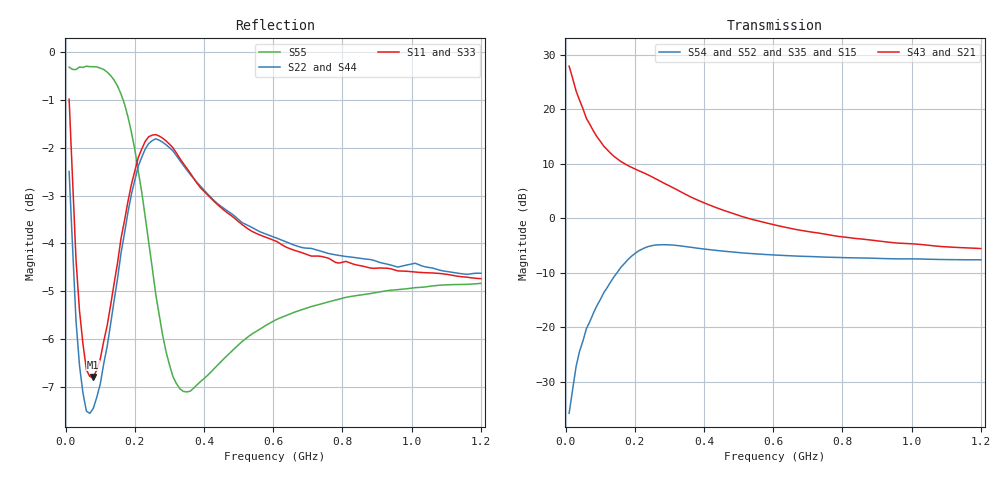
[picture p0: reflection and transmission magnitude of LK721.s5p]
! Date: Fri Jan 15 13:51:43 1999
!  POLYFET RF DEVICES
!  LK721 (EACH SIDE)
!  12.5Vdc		200ma
!AWR Design Environment (2053) Wed Feb 04 14:52:41 2004
!freq-unit  param-type  data-format  keyword  impedance-ohms
# MHz  S  MA  R  50
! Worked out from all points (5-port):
!   120 points, 10 MHz to 1.2 GHz, reference 50 ohm
!   strongest paths, dB at 10 MHz, 310 MHz, 610 MHz, 910 MHz, 1.2 GHz:
!     S43: 27.9, 5.6, -1.3, -4.2, -5.6
!     S21: 27.9, 5.6, -1.3, -4.2, -5.6
!     S54: -35.8, -4.9, -6.8, -7.4, -7.6
!     S52: -35.8, -4.9, -6.8, -7.4, -7.6
!     S35: -36.3, -5.0, -6.8, -7.4, -7.6
!     S15: -36.3, -5.0, -6.8, -7.4, -7.6
!   lowest |S11| = -6.8 dB at 80 MHz (marker M1), VSWR 2.68, Z = 53.1 - j52.9 ohm
!   |S11| at or under -10 dB: nowhere
